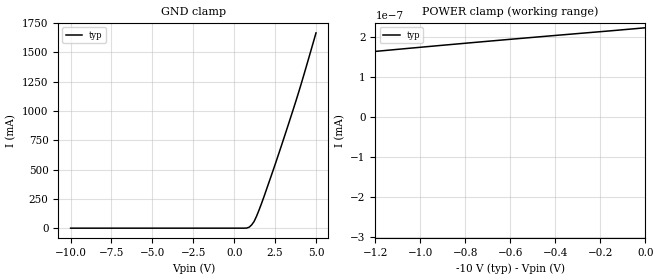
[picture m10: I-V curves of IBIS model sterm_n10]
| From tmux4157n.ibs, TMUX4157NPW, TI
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| sterm_n10
[Model]   sterm_n10
Model_type   Terminator
|   typ   min   max
C_comp   4.826588e-12   NA   NA
[Voltage Range]   -10   NA   NA
[Temperature Range]   27   NA   NA
[Power Clamp Reference]   -10   NA   NA
[GND Clamp Reference]   0   NA   NA
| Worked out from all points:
|   POWER clamp passes 1 mA (typ) near -10.76 V on its own axis
[GND Clamp]
|   Voltage   I(typ)   I(min)   I(max)
-10V      -794.2pA   NA         NA
606.1mV   76.38uA    NA         NA
909.1mV   7.912mA    NA         NA
1.061V    27.01mA    NA         NA
1.212V    56.16mA    NA         NA
1.364V    101.2mA    NA         NA
1.667V    209.5mA    NA         NA
2.273V    450.8mA    NA         NA
2.879V    701.4mA    NA         NA
3.788V    1.092A     NA         NA
4.242V    1.302A     NA         NA
5V        1.667A     NA         NA
[POWER Clamp]
|   Voltage   I(typ)   I(min)   I(max)
-15V      -1.828A    NA         NA
-6.818V   -297.4pA   NA         NA
-6.667V   -278.9pA   NA         NA
-6.212V   -225.9pA   NA         NA
-5.758V   -176.5pA   NA         NA
-5.152V   -115.8pA   NA         NA
-4.394V   -47.79pA   NA         NA
-3.636V   12.5pA     NA         NA
-2.879V   65.99pA    NA         NA
-1.97V    122.6pA    NA         NA
-1.061V   172.4pA    NA         NA
0V        224.4pA    NA         NA
